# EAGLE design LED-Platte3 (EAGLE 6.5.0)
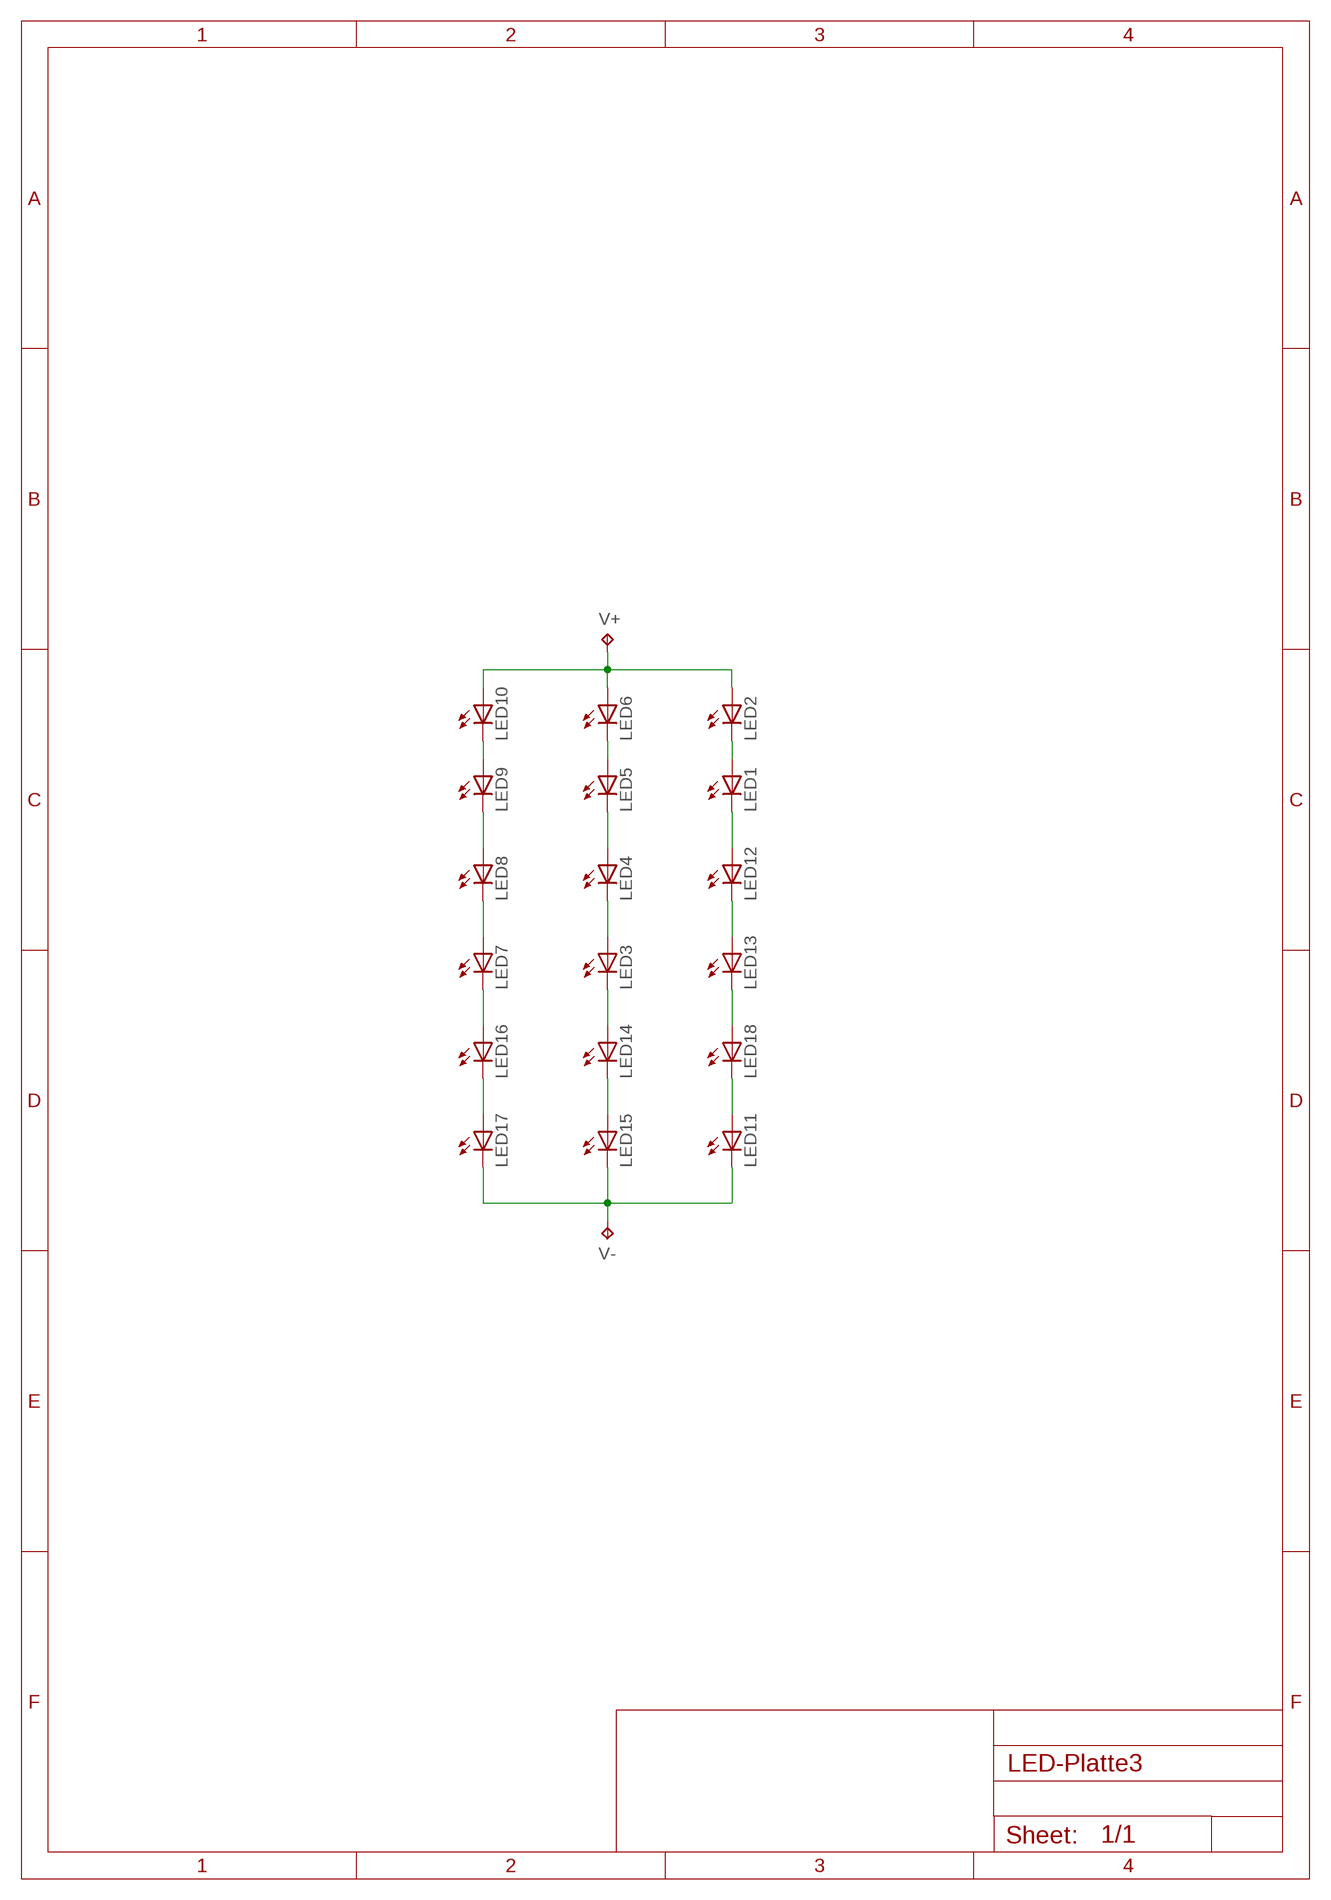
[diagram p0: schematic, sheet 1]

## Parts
LED1  LED-5630  [LED_5630]
LED2  LED-5630  [LED_5630]
LED3  LED-5630  [LED_5630]
LED4  LED-5630  [LED_5630]
LED5  LED-5630  [LED_5630]
LED6  LED-5630  [LED_5630]
LED7  LED-5630  [LED_5630]
LED8  LED-5630  [LED_5630]
LED9  LED-5630  [LED_5630]
LED10  LED-5630  [LED_5630]
LED11  LED-5630  [LED_5630]
LED12  LED-5630  [LED_5630]
LED13  LED-5630  [LED_5630]
LED14  LED-5630  [LED_5630]
LED15  LED-5630  [LED_5630]
LED16  LED-5630  [LED_5630]
LED17  LED-5630  [LED_5630]
LED18  LED-5630  [LED_5630]
V+  TPB2,54  [B2,54]
V-  TPB2,54  [B2,54]

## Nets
N$1: LED8.A1(A) LED8.A2(A) LED8.A3(A) LED9.C1(C) LED9.C2(C)
N$2: LED7.A1(A) LED7.A2(A) LED7.A3(A) LED8.C1(C) LED8.C2(C)
N$3: LED9.A1(A) LED9.A2(A) LED9.A3(A) LED10.C1(C) LED10.C2(C)
N$4: LED7.C1(C) LED7.C2(C) LED16.A1(A) LED16.A2(A) LED16.A3(A)
N$5: LED16.C1(C) LED16.C2(C) LED17.A1(A) LED17.A2(A) LED17.A3(A)
N$6: LED5.A1(A) LED5.A2(A) LED5.A3(A) LED6.C1(C) LED6.C2(C)
N$7: LED4.A1(A) LED4.A2(A) LED4.A3(A) LED5.C1(C) LED5.C2(C)
N$8: LED3.A1(A) LED3.A2(A) LED3.A3(A) LED4.C1(C) LED4.C2(C)
N$9: LED3.C1(C) LED3.C2(C) LED14.A1(A) LED14.A2(A) LED14.A3(A)
N$10: LED14.C1(C) LED14.C2(C) LED15.A1(A) LED15.A2(A) LED15.A3(A)
N$11: LED1.A1(A) LED1.A2(A) LED1.A3(A) LED2.C1(C) LED2.C2(C)
N$12: LED1.C1(C) LED1.C2(C) LED12.A1(A) LED12.A2(A) LED12.A3(A)
N$13: LED12.C1(C) LED12.C2(C) LED13.A1(A) LED13.A2(A) LED13.A3(A)
N$14: LED13.C1(C) LED13.C2(C) LED18.A1(A) LED18.A2(A) LED18.A3(A)
N$15: LED11.A1(A) LED11.A2(A) LED11.A3(A) LED18.C1(C) LED18.C2(C)
N$16: LED11.C1(C) LED11.C2(C) LED15.C1(C) LED15.C2(C) LED17.C1(C) LED17.C2(C) V-.TP
N$17: LED2.A1(A) LED2.A2(A) LED2.A3(A) LED6.A1(A) LED6.A2(A) LED6.A3(A) LED10.A1(A) LED10.A2(A) LED10.A3(A) V+.TP

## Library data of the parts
LED1-LED18 = Brunner:LED
V+ V- = testpad:TP: Test pad

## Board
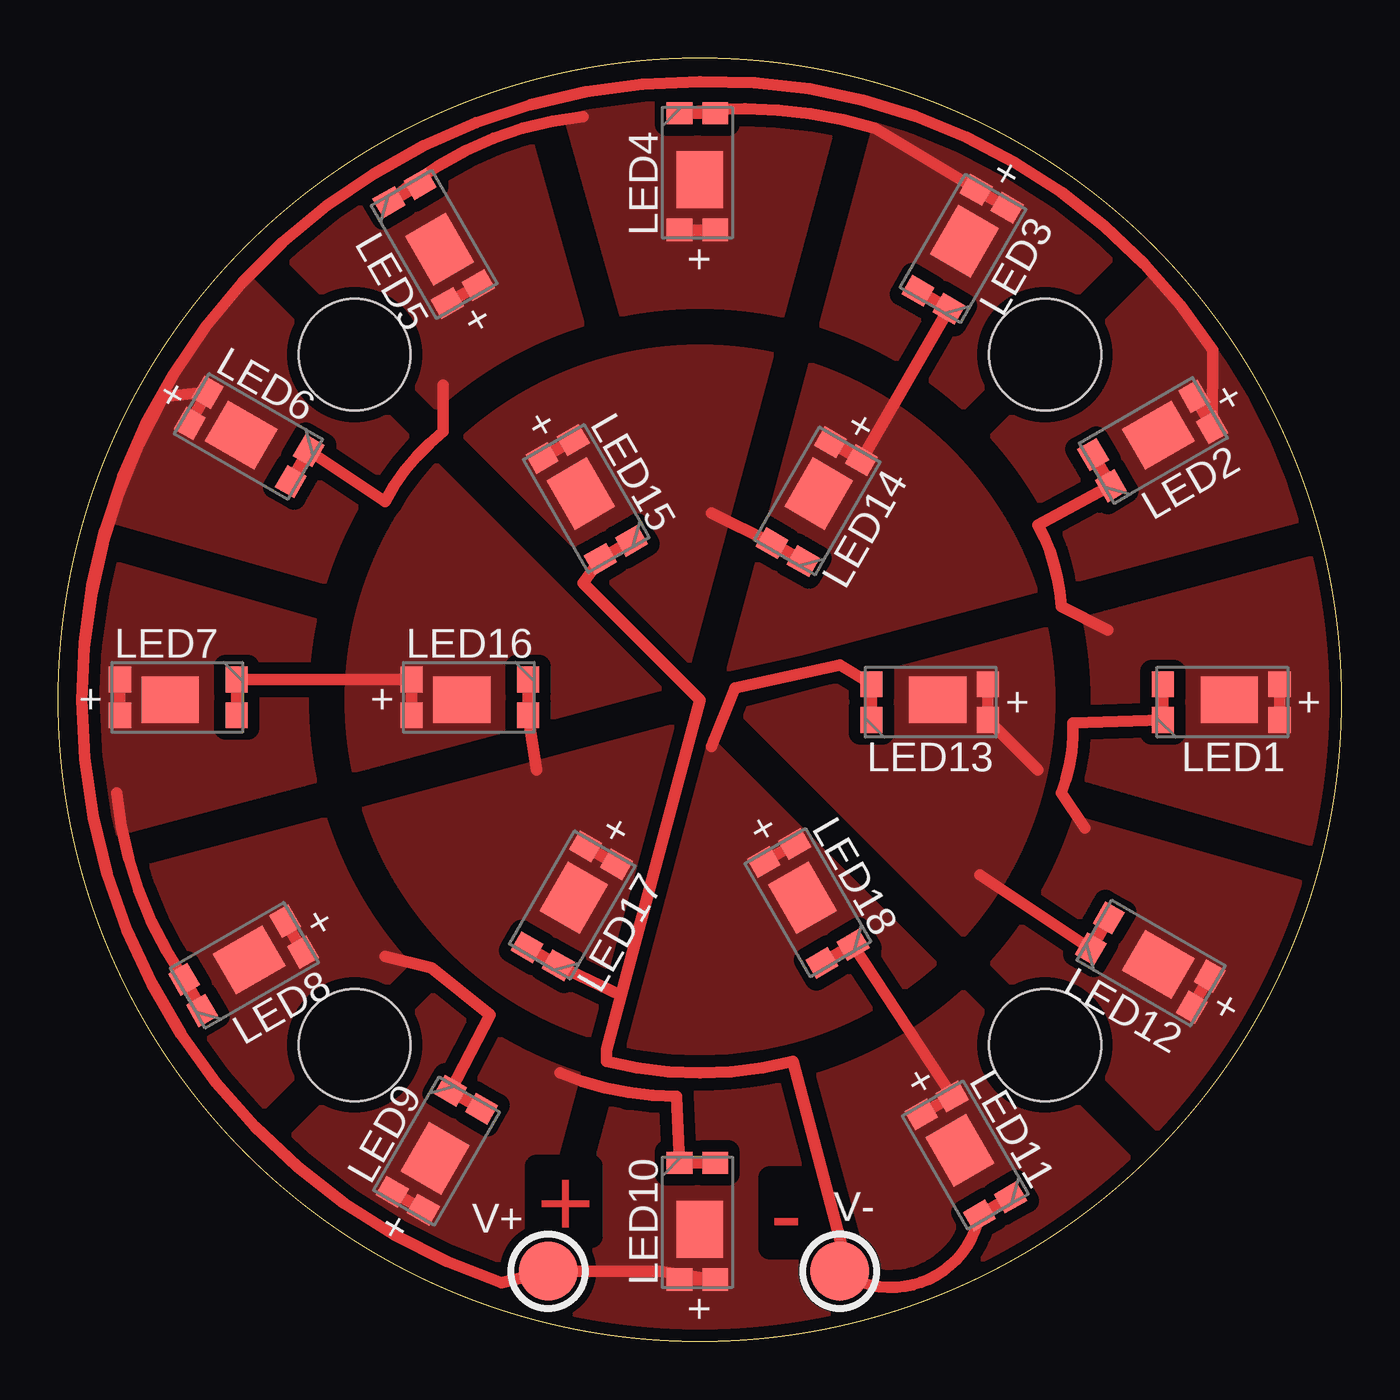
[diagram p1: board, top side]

Size 55 x 55 mm. Coordinates in mm from the lower left corner, seen from the top.
Outline: circle at 27.5,27.5 radius 27.5
Copper layers (1*16): Top 0.035mm / dielectric 1.5mm / Bottom 0.035mm
Design rules "default *": minimum track width 0.25mm, minimum drill 0.5mm, track to track 0.3mm, track to pad 0.3mm, pad to pad 0.3mm, via to via 0.3mm, smd to smd 8mil, copper to edge 0.5mm, drill to drill 0.3mm, minimum pad ring 10mil, minimum via ring 8mil, stop-mask expansion 4mil, vias tented up to drill 0mil, thermal gap 10mil
Holes 4.8 mm at 12.7,12.7 12.7,42.3 42.3,42.3 42.3,12.7
tRestrict: area 11.5,11.5 to 43.5,43.5; area 19.5,1.5 to 22.5,4.5; 12 lines

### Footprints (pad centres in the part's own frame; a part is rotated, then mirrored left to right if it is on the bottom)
LED_5630 = smd 0.95 x 1.1: A1 -2.36,0.87; A2 -2.36,-0.67; C1 2.64,0.87; C2 2.64,-0.67 | smd 2.45 x 2: A3 -0.2,0
B2,54 = smd 2.54 x 2.54: TP 0,0

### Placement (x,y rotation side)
LED1  50,27.5 180 top
LED2  46.99,38.75 210 top
LED3  38.75,46.99 240 top
LED4  27.5,50 90 top
LED5  16.25,46.99 120 top
LED6  8.01,38.75 330 top
LED7  5,27.5 0 top
LED8  8.01,16.25 210 top
LED9  16.25,8.01 60 top
LED10  27.5,5 90 top
LED11  38.75,8.01 300 top
LED12  46.99,16.25 150 top
LED13  37.5,27.5 180 top
LED14  32.5,36.16 240 top
LED15  22.5,36.16 300 top
LED16  17.5,27.5 0 top
LED17  22,18.84 240 top
LED18  32,18.84 300 top
U$1  [A4P-LOC]  not placed on the board
V+  21,3 0 top
V-  33.5,3 0 top

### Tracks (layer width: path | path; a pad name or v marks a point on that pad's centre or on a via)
N$1
  Top 0.5: LED8.A1 LED8.A2 | 14,16.5 16,16 18.5,14 LED9.C1 LED9.C2
  pour Top (isolate 0.5, no thermals): 6,5.5 0,20 12,24 16.5,16.5
N$2
  Top 0.5: LED7.A2 LED7.A1 | LED8.C1 LED8.C2 arc-29 2.5,23.5
  pour Top (isolate 0.5, no thermals): 0.5,20 0.5,35 13,32 12.5,23
N$3
  Top 0.5: LED9.A2 LED9.A1 | 21.5,11.5 arc23 26.5,10.5 LED10.C1 LED10.C2
  pour Top (isolate 0.5, no thermals): 22.96,11.83 19.96,-1.1 6.33,6.15 15.83,15.58
N$4
  Top 0.5: LED16.A2 LED16.A1 LED7.C1 LED7.C2
  pour Top (isolate 0.5, no thermals): 12,23.5 arc-56 16,39 26.5,28 26.5,27
N$5
  Top 0.5: LED17.A1 LED17.A2 | LED16.C1 LED16.C2 20.5,24.5
  pour Top (isolate 0.5, no thermals): 25.96,20.33 23.46,11.9 arc-53 11.83,23.15 27.33,27.58
N$6
  Top 0.5: LED5.A2 LED5.A1 | 16.5,41 16.5,39 arc23 14,36 LED6.C1 LED6.C2
  pour Top (isolate 0.5, no thermals): 16.6,38.42 6.6,48.35 19.73,56.1 24.23,43.67
N$7
  Top 0.5: LED4.A2 LED4.A1 | 22.5,52.5 arc36 LED5.C1 LED5.C2
  pour Top (isolate 0.5, no thermals): 23.5,42.5 20.5,55.5 36,56.5 32,42.5
N$8
  Top 0.5: LED3.A2 LED3.A1 35,52 arc25 LED4.C1 LED4.C2
  pour Top (isolate 0.5, no thermals): 49.46,49.33 38.96,38.4 31.33,42.65 35.33,56.58
N$9
  Top 0.5: LED14.A2 LED14.A1 LED3.C1 LED3.C2
  pour Top (isolate 0.5, no thermals): 42.96,31.33 28.46,28.4 27.33,27.65 31.83,43.08 arc-58
N$10
  Top 0.5: LED15.A1 LED15.A2 | LED14.C1 LED14.C2 28,35.5
  pour Top (isolate 0.5, no thermals): 26.6,27.92 16.1,38.85 arc-61 31.73,43.1 27.73,27.67
N$11
  Top 0.5: LED1.A2 LED1.A1 | 45,30.5 43,31.5 arc25 42,35 LED2.C1 LED2.C2
  pour Top (isolate 0.5, no thermals): 43,23.5 43,31.5 58.5,35.5 56.5,19.5
N$12
  Top 0.5: LED12.A2 LED12.A1 | 44,22 43,23.5 arc23 43.5,26.5 LED1.C1 LED1.C2
  pour Top (isolate 0.5, no thermals): 48.33,7.04 38.4,16.54 42.65,23.67 56.58,19.17
N$13
  Top 0.5: LED13.A2 LED13.A1 42,24.5 | 39.5,20 LED12.C1 LED12.C2
  pour Top (isolate 0.5, no thermals): 27.5,27.5 34.5,29.5 43,31.5 arc-56 39,16.5
N$14
  Top 0.5: LED18.A2 LED18.A1 | 28,25.5 29,28 33.5,29 LED13.C2 LED13.C1
  pour Top (isolate 0.5, no thermals): 23.1,11.92 25.5,20 27.73,27.1 39.23,16.17 arc-50
N$15
  Top 0.5: LED11.A2 LED11.A1 LED18.C1 LED18.C2
  pour Top (isolate 0.5, no thermals): 35.1,-2.08 32.1,11.85 38.73,16.6 49.23,6.17
N$16
  Top 0.5: 34,3.5 V-.TP 34,2.5 | 34,2.5 31.5,12 arc-29 23.5,12 23.5,12.5 24.12,14.83 | 34,2.5 34.5,2.5 arc97 LED11.C2 LED11.C1 | 24.12,14.83 27.5,27.5 22.5,32.5 LED15.C2 LED15.C1 | 24.12,14.83 LED17.C1 LED17.C2
N$17
  Top 0.5: 1,27.5 arc-90 27.5,54 arc-58 49.5,42.5 LED2.A1 LED2.A2 | 1,27.5 arc71 19,2.5 V+.TP 25.8,3 LED10.A2 LED10.A1 | LED6.A2 LED6.A1 4.5,40.5 arc29 1,27.5
  pour Top (isolate 0.5, no thermals): 12.33,30.54 1.9,34.54 arc-25 8.65,46.17 16.58,38.67
  pour Top (isolate 0.5, no thermals): 20,-1 23,12 31.5,12 34.5,-1
  pour Top (isolate 0.5, no thermals): 53.08,35.1 43.15,31.6 38.4,38.73 46.33,46.23 arc-31

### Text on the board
Top: + | -
tStop: + | -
